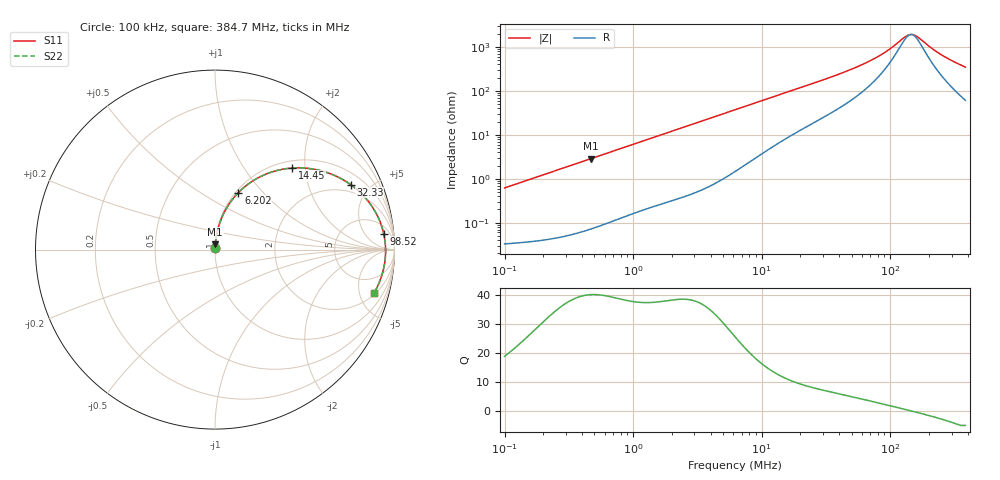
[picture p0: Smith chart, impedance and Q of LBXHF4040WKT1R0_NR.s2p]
! LBXHF4040WKT1R0_NR  S-PARAMETER MODEL  ( General Type )
! Model Generated by TAIYO YUDEN Corporation (http://www.ty-top.com)
! Version 1.0
! TAIYO YUDEN Control No. 210719NI43SB-FBB
! Copyright(c) 2021 TAIYO YUDEN CO.,LTD. All Rights Reserved.
! Product Description (link to TY-COMPAS)
! https://ds.yuden.co.jp/TYCOMPAS/or/detail?pn=LBXHF4040WKT1R0MNR&u=M
! Products Name : Inductors
! Characteristics :
!  Inductance : 1.0 uH , SRF(min) : 105 MHz , DC Resistance(max) : 0.031 Ohm
!  Rated Current : Saturation :4600 mA , Temp Rise : 2430 mA
!  Case Size : 4.0 x 4.0 / 0.157 x 0.157 [mm/inch] , Thickness : 2 / 0.079 [mm/inch]
!  (Conditions: Temperature = 25 degC , DC Bias Current/Voltage = 0A / 0V)
! External Node Assignments :
!  1  o---GGG---o  2
! GND o---------o GND
! Frequency Range : 0.1MHz  -  384.651195MHz  [ 402 STEP ]
# MHz S RI R 50
! Freq[MHz].  S11 Real  S11 Imag  S21 Real  S21 Imag  S12 Real  S12 Imag  S22 Real  S22 Imag
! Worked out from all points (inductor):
!   401 points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, 100 kHz to 384.7 MHz, reference 50 ohm
!   read as one part in series: L = 982 nH near 104.2 kHz
!   highest Q = 40 at 470.1 kHz (marker M1), where L = 975 nH
!   self-resonance near 145.5 MHz
!   S11 on the Smith chart (normalised r, x): 100 kHz: 1.00, +0.01; 6.202 MHz: 1.03, +0.74; 14.45 MHz: 1.15, +1.71; 32.33 MHz: 1.56, +3.79; 98.52 MHz: 9, +15; 384.7 MHz: 2.22, -6.84
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0.1  0.000367 0.00618  0.9996 -0.00618  0.9996 -0.00618  0.000367 0.00618
0.398565  0.00121 0.0244  0.9988 -0.0244  0.9988 -0.0244  0.00121 0.0244
0.470111  0.00155 0.0287  0.9985 -0.0287  0.9985 -0.0287  0.00155 0.0287
1.588538  0.0115 0.0943  0.9885 -0.0943  0.9885 -0.0943  0.0115 0.0943
3.552561  0.0483 0.201  0.9517 -0.201  0.9517 -0.201  0.0483 0.201
6.202025  0.1306 0.3179  0.8694 -0.3179  0.8694 -0.3179  0.1306 0.3179
6.331348  0.1353 0.3226  0.8647 -0.3226  0.8647 -0.3226  0.1353 0.3226
9.17961  0.2438 0.402  0.7562 -0.402  0.7562 -0.402  0.2438 0.402
14.45449  0.4303 0.4544  0.5697 -0.4544  0.5697 -0.4544  0.4303 0.4544
24.71908  0.6612 0.4153  0.3388 -0.4153  0.3388 -0.4153  0.6612 0.4153
32.32563  0.7553 0.3626  0.2447 -0.3626  0.2447 -0.3626  0.7553 0.3626
61.29001  0.8969 0.204  0.1031 -0.204  0.1031 -0.204  0.8969 0.204
78.51302  0.9245 0.1426  0.0755 -0.1426  0.0755 -0.1426  0.9245 0.1426
98.5215  0.9401 0.0888  0.0599 -0.0888  0.0599 -0.0888  0.9401 0.0888
134.2675  0.9498 0.0182  0.0502 -0.0182  0.0502 -0.0182  0.9498 0.0182
142.843  0.9504 0.0042  0.0496 -0.0042  0.0496 -0.0042  0.9504 0.0042
151.9662  0.9505 -0.00977  0.0495 0.00977  0.0495 0.00977  0.9505 -0.00977
165.0432  0.95 -0.0285  0.05 0.0285  0.05 0.0285  0.95 -0.0285
211.4218  0.9436 -0.0858  0.0564 0.0858  0.0564 0.0858  0.9436 -0.0858
249.3739  0.9347 -0.1257  0.0653 0.1257  0.0653 0.1257  0.9347 -0.1257
312.9251  0.915 -0.1836  0.085 0.1836  0.085 0.1836  0.915 -0.1836
384.6512  0.8874 -0.2394  0.1126 0.2394  0.1126 0.2394  0.8874 -0.2394
